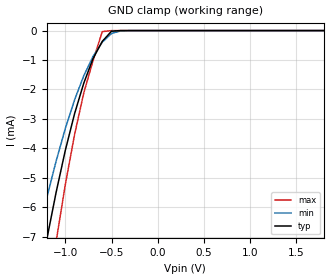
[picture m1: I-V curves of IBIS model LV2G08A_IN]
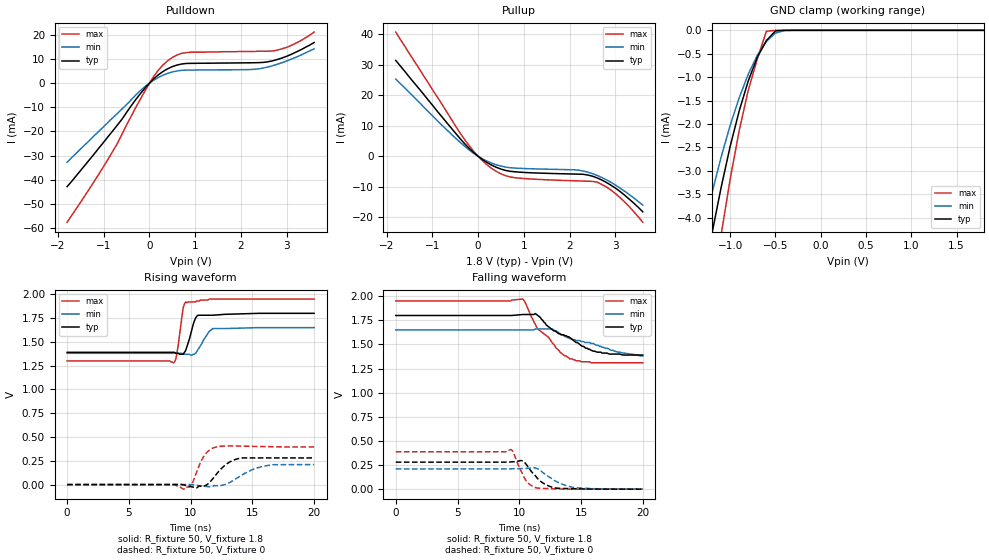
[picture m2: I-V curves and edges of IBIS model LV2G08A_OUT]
|/_/_/_/_/_/_/_/_/_/_/_/_/_/_/_/_/_/_/_/_/_/_/_/_/_/_/_/_/_/_/_/_/_/_/_/_/_/
|   Renesas Electronics Corp.
|   Multi Purpose Semiconductor Digital IC Design Group
|   IBIS Model of HD74LV2G08A
|   1.8V Dual 2-input AND Gates,  SSOP-8(8pin) Package
|   History
|   V1.0   April   1, 2003   : First release.
|/_/_/_/_/_/_/_/_/_/_/_/_/_/_/_/_/_/_/_/_/_/_/_/_/_/_/_/_/_/_/_/_/_/_/_/_/_/
[IBIS Ver]   2.1
[Comment Char]  |_char
[File name]   l2g08s1.ibs
[File Rev]   1.1
[Date]   April 1, 2003
[Source]   Data created from SPICE simulations at
|   Renesas Electronics Corp.
[Notes]   RLC value of the Package is determined by assuming typical
|   conditions.
[Disclaimer]   This information is for modeling purposes only, and is not
|   guaranteed.
[Copyright]   Copyright 2003, Renesas Electronics Corp.,
|   All Rights Reserved.
|   Component  HD74LV2G08A
[Component]   HD74LV2G08A
[Manufacturer]  Renesas Electronics Corp.
[Package]
|   typ   min   max
R_pkg   0.099   0.095   0.102
L_pkg   1.740nH   1.680nH   1.790nH
C_pkg   0.140pF   0.140pF   0.150pF
[Pin]   signal_name   model_name   R_pin   L_pin   C_pin
1   1A   LV2G08A_IN   0.102   1.780nH   0.140pF
2   1B   LV2G08A_IN   0.097   1.710nH   0.150pF
3   2Y   LV2G08A_OUT   0.095   1.680nH   0.150pF
4   GND   GND   0.102   1.790nH   0.140pF
5   2A   LV2G08A_IN   0.101   1.790nH   0.140pF
6   2B   LV2G08A_IN   0.097   1.710nH   0.150pF
7   1Y   LV2G08A_OUT   0.097   1.710nH   0.150pF
8   VCC   POWER   0.102   1.790nH   0.140pF
| Models and submodels in the file (2): LV2G08A_IN (Input), LV2G08A_OUT (Output)
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|   Model  LV2G08A_IN
[Model]   LV2G08A_IN
Model_type  Input
Vinl = 0.54V
Vinh = 1.26V
| variable   typ   min   max
C_comp   2.35pF   2.25pF   2.45pF
| variable   typ   min   max
[Temperature range]   25   85   -40
| variable   typ   min   max
[Voltage range]   1.8V   1.65V   1.95V
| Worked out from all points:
|   GND clamp passes 1 mA (typ) near -0.71 V on its own axis
[GND Clamp]
|   Voltage   I(typ)   I(min)   I(max)
-1.8V     -19.4mA    -15.4mA    -25.6mA
-1.3V     -8.81mA    -7.02mA    -11.6mA
-1.2V     -7.07mA    -5.66mA    -9.31mA
-1.1V     -5.49mA    -4.43mA    -7.16mA
-1V       -4.06mA    -3.32mA    -5.22mA
-900mV    -2.82mA    -2.35mA    -3.53mA
-800mV    -1.78mA    -1.53mA    -2.11mA
-700mV    -950uA     -877uA     -1.02mA
-600mV    -366uA     -393uA     -35.6uA
-500mV    -21.6uA    -99uA      -429nA
-400mV    -422nA     -10.2uA    -2.45nA
1.8V      3.69pA     25.5pA     3.6pA
|   Model  LV2G08A_OUT
[Model]   LV2G08A_OUT
Model_type  Output
Polarity   Inverting
| variable   typ   min   max
C_comp   4.85pF   4.75pF   4.95pF
| variable   typ   min   max
[Temperature range]   25   85   -40
| variable   typ   min   max
[Voltage range]   1.8V   1.65V   1.95V
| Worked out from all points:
|   slope of the pulldown table from 0 to 0.27 V, typ, clamps not added: 60.6 ohm
|   slope of the pullup table from 0 to 0.27 V, typ, clamps not added: 101 ohm
|   GND clamp passes 1 mA (typ) near -0.78 V on its own axis
|   rising waveform, R_fixture 50, V_fixture 1.8: 20-80 % time 540ps typ, 760ps min, 406ps max; typ from 1.39 V to 1.8 V
|   rising waveform, R_fixture 50, V_fixture 0: 20-80 % time 1.24ns typ, 1.8ns min, 830ps max; typ from 0 V to 0.28 V
|   falling waveform, R_fixture 50, V_fixture 1.8: 20-80 % time 3.17ns typ, 4.12ns min, 2.35ns max; typ from 1.8 V to 1.39 V
|   falling waveform, R_fixture 50, V_fixture 0: 20-80 % time 1.27ns typ, 1.73ns min, 877ps max; typ from 0.28 V to 0 V
[Pullup]
|   Voltage   I(typ)   I(min)   I(max)
-1.8V     31.4mA     25.3mA     40.7mA
-400mV    5.92mA     4.69mA     7.77mA
-100mV    1.26mA     991uA      1.71mA
200mV     -2.09mA    -1.62mA    -2.86mA
500mV     -4.2mA     -3.22mA    -5.75mA
800mV     -5.08mA    -3.86mA    -7.01mA
2.1V      -5.82mA    -4.43mA    -8.04mA
2.4V      -6.15mA    -5.21mA    -8.18mA
2.6V      -7.07mA    -6.27mA    -8.47mA
2.9V      -9.44mA    -8.5mA     -11mA
3.1V      -11.5mA    -10.4mA    -13.5mA
3.6V      -18.2mA    -16mA      -21.6mA
[Pulldown]
|   Voltage   I(typ)   I(min)   I(max)
-1.8V     -42.8mA    -32.7mA    -57.5mA
-900mV    -22mA      -16.1mA    -31.3mA
-700mV    -17.3mA    -12.5mA    -24.9mA
-100mV    -2.12mA    -1.47mA    -3.28mA
100mV     1.89mA     1.29mA     2.99mA
400mV     5.95mA     4.05mA     9.28mA
600mV     7.46mA     5.03mA     11.6mA
900mV     8.17mA     5.4mA      12.8mA
2.2V      8.4mA      5.62mA     13.1mA
2.6V      8.86mA     6.72mA     13.2mA
3V        11.1mA     9.16mA     14.8mA
3.6V      16.8mA     14.2mA     21.1mA
[GND Clamp]
|   Voltage   I(typ)   I(min)   I(max)
-1.8V     -11.9mA    -9.46mA    -15.7mA
-1.3V     -5.4mA     -4.31mA    -7.13mA
-1.2V     -4.33mA    -3.47mA    -5.69mA
-1.1V     -3.36mA    -2.71mA    -4.37mA
-1V       -2.48mA    -2.03mA    -3.18mA
-900mV    -1.72mA    -1.44mA    -2.14mA
-800mV    -1.08mA    -936uA     -1.28mA
-700mV    -575uA     -533uA     -610uA
-600mV    -219uA     -237uA     -20.5uA
-500mV    -12.9uA    -58.6uA    -245nA
-400mV    -248nA     -6.13uA    -1.4nA
1.8V      1.91pA     29.2pA     1.8pA
[Ramp]
| variable   typ   min   max
dV/dt_r   0.171/1.274n   0.131/1.925n   0.233/807.0p
dV/dt_f   0.246/3.165n   0.157/3.956n   0.386/2.342n
R_load = 50ohms
[Rising Waveform]
R_fixture = 50
V_fixture = 1.8
V_fixture_min = 1.65
V_fixture_max = 1.95
C_fixture = 0p
|   Time   V(typ)   V(min)   V(max)
0s        1.39V      1.38V      1.3V
8.6ns     1.39V      1.38V      1.28V
8.8ns     1.38V      1.38V      1.32V
9ns       1.38V      1.38V      1.47V
9.4ns     1.37V      1.37V      1.86V
9.6ns     1.41V      1.37V      1.92V
10.3ns    1.72V      1.37V      1.92V
10.6ns    1.78V      1.42V      1.93V
11.8ns    1.78V      1.64V      1.95V
20ns      1.8V       1.65V      1.95V
[Rising Waveform]
R_fixture = 50
V_fixture = 0
C_fixture = 0p
|   Time   V(typ)   V(min)   V(max)
0s        242pV      529nV      109pV
8.7ns     242pV      529nV      109pV
9.4ns     -2.85mV    606uV      -48.3mV
10ns      -20.7mV    485uV      -16mV
11ns      -18.1mV    -15.8mV    283mV
11.9ns    78.6mV     -9.35mV    388mV
12.9ns    215mV      6.38mV     406mV
14ns      277mV      88.3mV     405mV
16.1ns    280mV      198mV      399mV
20ns      280mV      210mV      395mV
[Falling Waveform]
R_fixture = 50
V_fixture = 1.8
V_fixture_min = 1.65
V_fixture_max = 1.95
C_fixture = 0p
|   Time   V(typ)   V(min)   V(max)
0s        1.8V       1.65V      1.95V
10.3ns    1.81V      1.65V      1.97V
11.5ns    1.8V       1.66V      1.66V
12.4ns    1.68V      1.66V      1.57V
12.7ns    1.65V      1.66V      1.51V
13.3ns    1.61V      1.61V      1.42V
14.1ns    1.57V      1.56V      1.35V
15.1ns    1.48V      1.53V      1.32V
16.3ns    1.42V      1.49V      1.31V
20ns      1.39V      1.38V      1.31V
[Falling Waveform]
R_fixture = 50
V_fixture = 0
C_fixture = 0p
|   Time   V(typ)   V(min)   V(max)
0s        280mV      210mV      387mV
9ns       280mV      210mV      387mV
9.3ns     282mV      210mV      411mV
9.5ns     284mV      211mV      386mV
10.3ns    291mV      214mV      151mV
10.7ns    233mV      217mV      65.6mV
11.3ns    140mV      220mV      16.8mV
12.5ns    27.1mV     120mV      4.9mV
14.4ns    4.17mV     17.3mV     105uV
20ns      -164uV     30.8uV     -95.4uV
